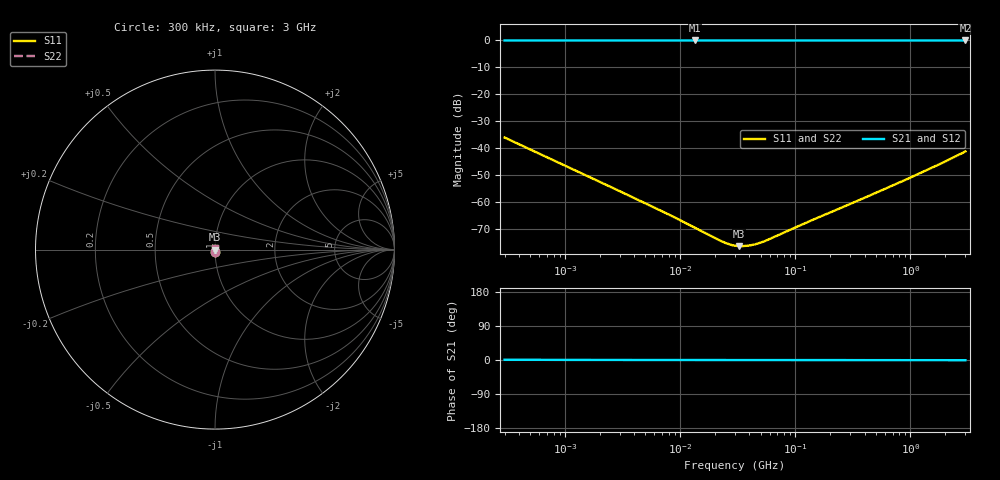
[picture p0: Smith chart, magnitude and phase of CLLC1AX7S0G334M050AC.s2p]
! S-Parameter Data Generated by TDK Corporation
! Copyright(C) 2024 TDK Corporation.
! All Rights Reserved.
! TDK P/N: CLLC1AX7S0G334M050AC (Multilayer Ceramic Chip Capacitor)
! Property: C=330nF
! Size(LxWxT): 1.6x0.8x0.5mm
! Model Type: s2p (Touchstone File Format Version 1.0)
! Frequency: DC=Yes Start=0.3MHz Stop=3000MHz 402points Log-sweep
! Model Generated on May 28, 2024
! Terms and conditions regarding TDK Simulation Models:
! 1)This simulation model is being provided solely for informational
!  purposes. Please refer to the specifications of the products in
!  terms of detailed characteristics of such products.
! 2)In no event shall TDK Corporation of any of its subsidiaries be
!  liable for any loss or damage arising, directly or indirectly,
!  from any information contained in this simulation model, including,
!  but not limited to loss or damages arising from any inaccuracies,
!  omissions or errors in connection with such information.
! 3)Any and all copyrights on this simulation model are owned by
!  TDK Corporation.  Duplication or redistribution of this simulation
!  model without prior written permission from TDK Corporation
!  is prohibited.
! 4)This simulation model is subject to any modification or change
!  without any prior notice.
! 5)Neither TDK Corporation nor any of its subsidiaries shall make any
!  warranty, express or implied, including but not limited to the
!  correctness, implied warranties of merchantability and fitness for
!  a particular purpose with respect to this simulation models.
! 6)The use of this simulation model shall be deemed to have consented
!  to the terms and conditions hereof.
! Port Assignments:
!  1 ---| |--- 2
! Applicable Conditions:
!  Temperature = 25 degC
!  DC Bias Voltage = 0 V
!  Small Signal Operation
# Hz S MA R 50
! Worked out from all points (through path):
!   401 points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, 300 kHz to 3 GHz, reference 50 ohm
!   highest |S21| = 0.00 dB at 13.55 MHz (marker M1); lowest = 0.0 dB at 3 GHz (marker M2)
!   lowest |S11| = -76.2 dB at 32.45 MHz (marker M3), VSWR 1.00, Z = 50 - j0.00274 ohm
!   |S11| at or under -10 dB: start of sweep to end of sweep
!   |S22| runs from -76.2 to -36.0 dB; largest |S21 - S12| = 0
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300000  0.01594 -88.1  0.9996 0.9  0.9996 0.9  0.01594 -88.1
316106  0.01513 -88.1  0.9996 0.9  0.9996 0.9  0.01513 -88.1
1417447  0.003411 -87.0  0.9998 0.2  0.9998 0.2  0.003411 -87.0
6477617  0.000743 -78.9  0.9999 0.0  0.9999 0.0  0.000743 -78.9
9171552  0.0005167 -74.0  0.9999 0.0  0.9999 0.0  0.0005167 -74.0
1.354884e7  0.0003374 -65.3  0.9999 0.0  0.9999 0.0  0.0003374 -65.3
2.173308e7  0.0002015 -43.9  0.9999 0.0  0.9999 0.0  0.0002015 -43.9
2.581679e7  0.0001732 -30.8  0.9999 0.0  0.9999 0.0  0.0001732 -30.8
2.756695e7  0.0001653 -25.0  0.9999 0.0  0.9999 0.0  0.0001653 -25.0
3e7  0.0001584 -17.7  0.9998 0.0  0.9998 0.0  0.0001584 -17.7
3.244533e7  0.0001551 -10.2  0.9998 0.0  0.9998 0.0  0.0001551 -10.2
3.570576e7  0.000156 -1.1  0.9998 0.0  0.9998 0.0  0.000156 -1.1
3.978131e7  0.00016 8.4  0.9998 -0.0  0.9998 -0.0  0.00016 8.4
4.465116e7  0.0001672 18.1  0.9998 -0.0  0.9998 -0.0  0.0001672 18.1
5.147625e7  0.0001837 28.9  0.9998 -0.0  0.9998 -0.0  0.0001837 28.9
6.006555e7  0.0002109 38.5  0.9998 -0.0  0.9998 -0.0  0.0002109 38.5
1.416118e8  0.0004751 64.9  0.9998 -0.0  0.9998 -0.0  0.0004751 64.9
6.485268e8  0.001919 79.3  0.9996 -0.1  0.9996 -0.1  0.001919 79.3
1.446734e9  0.004128 81.5  0.9994 -0.2  0.9994 -0.2  0.004128 81.5
1.831088e9  0.005224 81.8  0.9993 -0.3  0.9993 -0.3  0.005224 81.8
2.880605e9  0.008415 80.5  0.9986 -0.5  0.9986 -0.5  0.008415 80.5
3e9  0.008824 80.1  0.9985 -0.5  0.9985 -0.5  0.008824 80.1
